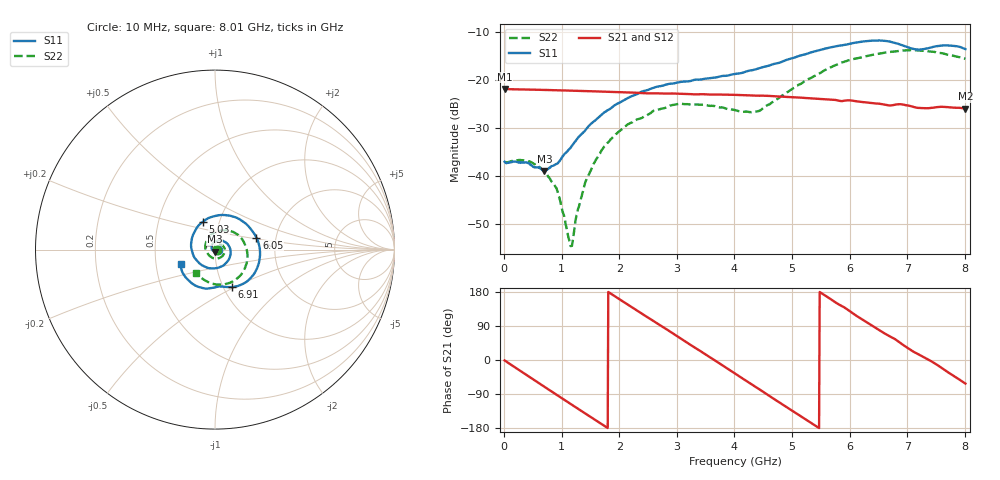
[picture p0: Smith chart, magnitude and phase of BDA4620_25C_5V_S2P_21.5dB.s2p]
!Agilent Technologies,E5071B,MY42404982,A.09.10
!Date: Wed May 06 09:02:59 2026
!Data & Calibration Information:
!Freq	S11:SOLT2(ON)	S21:SOLT2(ON)	S12:SOLT2(ON)	S22:SOLT2(ON)
# Hz S RI R 50
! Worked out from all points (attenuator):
!   801 points, 10 MHz to 8.01 GHz, reference 50 ohm
!   highest |S21| = -21.91 dB at 10 MHz (marker M1); lowest = -26.0 dB at 8.01 GHz (marker M2)
!   lowest |S11| = -39.0 dB at 700 MHz (marker M3), VSWR 1.02, Z = 49.8 - j1.1 ohm
!   |S11| at or under -10 dB: start of sweep to end of sweep
!   |S22| runs from -54.6 to -13.8 dB; largest |S21 - S12| = 0.0004
!   S11 on the Smith chart (normalised r, x): 10 MHz: 1.03, -0.00; 5.03 GHz: 0.83, +0.27; 6.05 GHz: 1.58, +0.23; 6.91 GHz: 1.10, -0.48; 8.01 GHz: 0.67, -0.12
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1e7  0.014 -0.000942  0.0803 -0.00169  0.0803 -0.00171  0.0137 -0.000462
4.3e8  0.0085 -0.0105  0.0574 -0.0544  0.0574 -0.0546  0.0133 -0.00495
7e8  -0.00213 -0.011  0.0261 -0.074  0.0262 -0.0741  0.00879 -0.00684
9.3e8  -0.0123 -0.00544  -0.00463 -0.0777  -0.00477 -0.0778  0.00336 -0.00599
1.15e9  -0.0184 0.0061  -0.033 -0.0698  -0.0331 -0.0698  -0.00144 -0.00121
1.19e9  -0.019 0.00886  -0.0377 -0.0671  -0.0378 -0.0672  -0.00207 6.38e-05
1.35e9  -0.0189 0.0199  -0.0543 -0.0539  -0.0544 -0.054  -0.00366 0.005
1.53e9  -0.0133 0.0331  -0.0676 -0.0345  -0.0677 -0.0346  -0.00342 0.0117
1.77e9  0.00269 0.0468  -0.075 -0.00451  -0.0751 -0.00449  0.000902 0.021
2.15e9  0.0415 0.0495  -0.0613 0.0413  -0.0613 0.0415  0.0176 0.0296
2.68e9  0.0852 0.00231  -0.00584 0.0719  -0.00577 0.0721  0.0451 0.0192
3.07e9  0.0767 -0.0564  0.0395 0.0599  0.0397 0.0597  0.0559 -0.00709
4.01e9  -0.0819 -0.0806  0.0566 -0.0407  0.0566 -0.0408  -0.0114 -0.0471
4.42e9  -0.1315 0.00439  0.0165 -0.0663  0.0165 -0.0664  -0.0458 -0.0125
5.03e9  -0.0677 0.1553  -0.0478 -0.0452  -0.0478 -0.0454  -0.0283 0.077
5.35e9  0.0282 0.1924  -0.0625 -0.0134  -0.0626 -0.0134  0.0234 0.1035
6.05e9  0.2311 0.0671  -0.0335 0.0505  -0.0336 0.0506  0.1552 0.0519
6.37e9  0.2469 -0.0633  -0.00265 0.0572  -0.00259 0.0572  0.1797 -0.0164
6.68e9  0.1769 -0.1782  0.0238 0.0486  0.0239 0.0487  0.1706 -0.0916
6.91e9  0.094 -0.2091  0.0413 0.0369  0.0415 0.037  0.1431 -0.1422
7.57e9  -0.0812 -0.2107  0.0497 -0.0163  0.0498 -0.0162  -0.0169 -0.1892
8.01e9  -0.1917 -0.0824  0.0232 -0.0442  0.0234 -0.0443  -0.1047 -0.1278
